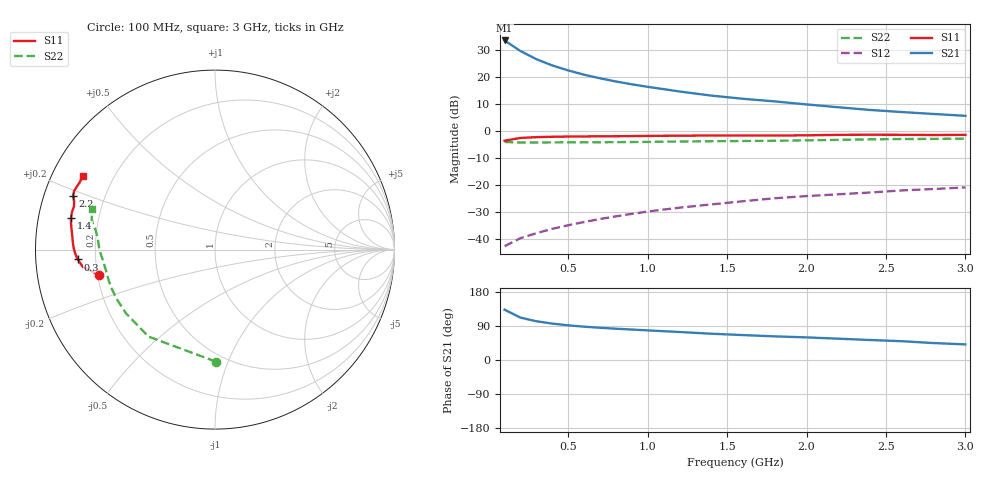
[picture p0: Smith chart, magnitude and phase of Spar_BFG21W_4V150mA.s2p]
! Filename: 4150bfg21.001
! Title: BFG21W
! Bias: Vce=4V; Ic=150mA
! Company: NXP Semiconductors NL
! User: Quality&Reliability T&D
! Measure time: 10 Nov 1999 / 11:46:10
#  MHz  S  MA  R 50
! Freq  S11  S21  S12  S22  :
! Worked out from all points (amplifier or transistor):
!   20 points, 100 MHz to 3 GHz, reference 50 ohm
!   highest |S21| = 33.5 dB at 100 MHz (marker M1)
!   |S21| within 3 dB of that: start of sweep to 176.6 MHz
!   unconditionally stable (mu >= 1): 587.4 MHz to end of sweep
!   at 400 MHz: K = 0.92, MSG = 30.2 dB, |S12| = -36.2 dB
!   at 1.2 GHz: K = 1.06, MAG = 20.0 dB, |S12| = -28.4 dB
!   at 3 GHz: K = 1.05, MAG = 11.9 dB, |S12| = -20.9 dB
!   S11 on the Smith chart (normalised r, x): 100 MHz: 0.21, -0.10; 300 MHz: 0.13, -0.04; 1.4 GHz: 0.10, +0.11; 2.2 GHz: 0.09, +0.18; 3 GHz: 0.09, +0.26
100  0.6592 -167.7  47.22 132.7  0.007365 56.5  0.6246 -89.5
200  0.7417 -172.4  30.07 111.9  0.01037 54.8  0.61 -127.4
300  0.7672 -175.9  21.24 102.2  0.01279 58.6  0.6099 -144.3
400  0.7789 -178.4  16.28 96.1  0.01541 62.1  0.6133 -153.6
500  0.7865 179.7  13.15 91.5  0.01796 65.0  0.6155 -159.6
600  0.7911 177.9  10.97 88.0  0.02061 67.0  0.6167 -163.8
700  0.7946 176.3  9.421 85.1  0.02343 68.9  0.6175 -167.0
800  0.7982 174.8  8.222 82.5  0.02624 70.2  0.6192 -169.8
900  0.8023 173.3  7.292 80.4  0.02912 71.6  0.6226 -172.2
1000  0.8073 172.0  6.547 78.2  0.03224 72.1  0.6265 -174.3
1200  0.816 169.5  5.37 73.9  0.03803 73.0  0.6366 -177.7
1400  0.8215 167.6  4.508 69.4  0.04359 73.1  0.6452 179.5
1600  0.8239 165.3  3.933 65.8  0.04995 73.2  0.6498 176.9
1800  0.8216 162.9  3.518 62.4  0.05674 73.1  0.6576 174.3
2000  0.8297 161.1  3.094 59.7  0.0622 73.5  0.6695 171.5
2200  0.8452 159.2  2.741 56.3  0.06719 73.2  0.684 169.3
2400  0.8502 157.4  2.443 52.7  0.07249 72.3  0.6986 167.6
2600  0.8463 155.6  2.235 49.6  0.07921 71.1  0.7081 166.1
2800  0.8412 153.3  2.059 44.7  0.08415 69.3  0.7124 164.1
3000  0.8456 150.8  1.905 41.2  0.09 68.3  0.7194 161.7
